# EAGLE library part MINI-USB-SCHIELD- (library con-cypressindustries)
MINI USB-B Conector Source: www.cypressindustries.com
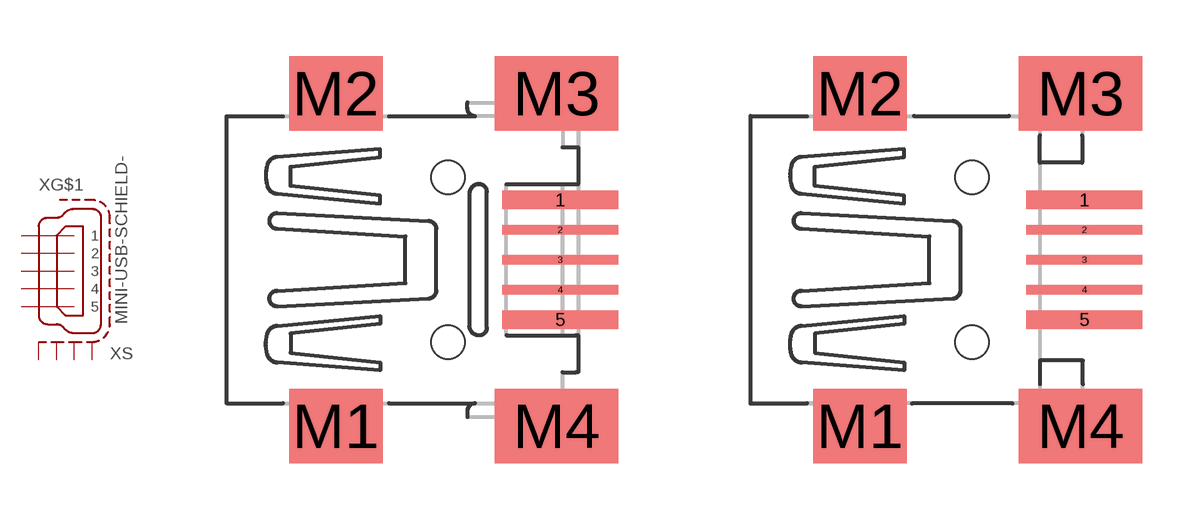
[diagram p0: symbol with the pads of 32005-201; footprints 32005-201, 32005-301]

Designator prefix X; gates G$1=MINI-USB-5 S=SHIELD_4

## MINI-USB-SCHIELD-32005-201 (OC_FARNELL: unknown; OC_NEWARK: unknown)  [32005-201]
1  G$1:1  pas
2  G$1:2  pas
3  G$1:3  pas
4  G$1:4  pas
5  G$1:5  pas
M1  S:S1  pas
M2  S:S2  pas
M3  S:S3  pas
M4  S:S4  pas

## MINI-USB-SCHIELD-32005-301 (OC_FARNELL: unknown; OC_NEWARK: unknown)  [32005-301]
Pads as for 32005-201

## Footprint 32005-201 (pad centres in mm)
MINI USB-B R/A SMT W/ REAR Source: http://www.cypressindustries.com/pdf/32005-201.pdf
smd 3.1 x 0.5: 1 3,1.6; 5 3,-1.6
smd 3.1 x 0.254: 2 3,0.8; 3 3,0; 4 3,-0.8
smd 2.5 x 2: M1 -3,-4.45; M2 -3,4.45
smd 3.3 x 2: M3 2.9,4.45; M4 2.9,-4.45
hole 0.9 at 0,2.2
hole 0.9 at 0,-2.2

## Footprint 32005-301 (pad centres in mm)
MINI USB-B R/A SMT W/O REAR Source: http://www.cypressindustries.com/pdf/32005-301.pdf
smd 3.1 x 0.5: 1 3,1.6; 5 3,-1.6
smd 3.1 x 0.254: 2 3,0.8; 3 3,0; 4 3,-0.8
smd 2.5 x 2: M1 -3,-4.45; M2 -3,4.45
smd 3.3 x 2: M3 2.9,4.45; M4 2.9,-4.45
hole 0.9 at 0,2.2
hole 0.9 at 0,-2.2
